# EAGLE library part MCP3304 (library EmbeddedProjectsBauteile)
Microchip 13-Bit Differential Input, Low Power A/D Converter with SPI Serial Interface
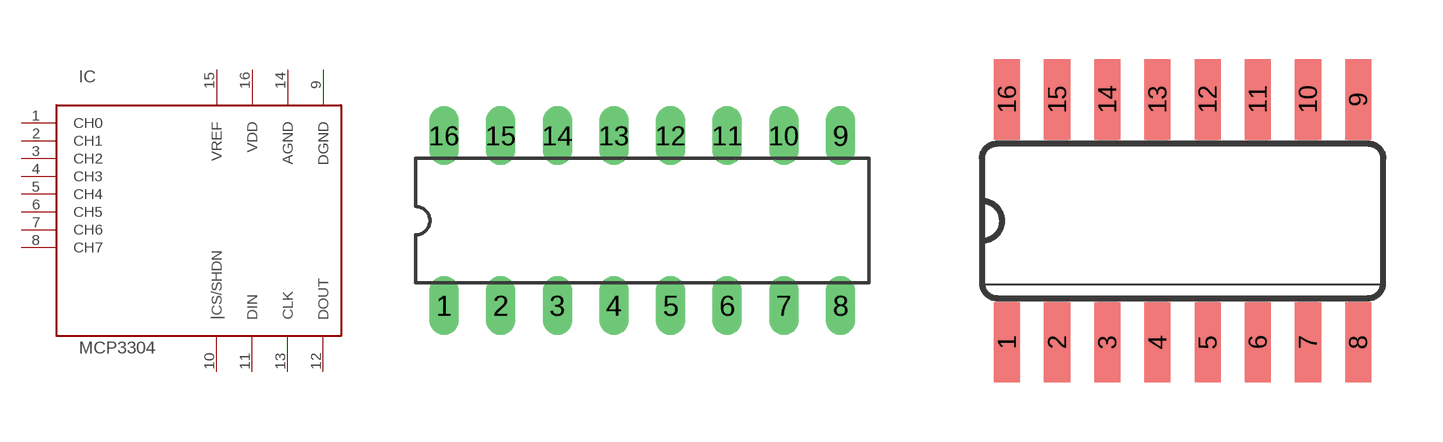
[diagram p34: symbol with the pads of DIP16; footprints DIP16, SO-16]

Designator prefix IC

## MCP3304BI/P (FARNELL: 1852025)  [DIP16]
1  CH0
2  CH1
3  CH2
4  CH3
5  CH4
6  CH5
7  CH6
8  CH7
9  DGND
10  |CS/SHDN
11  DIN
12  DOUT
13  CLK
14  AGND
15  VREF
16  VDD

## MCP3304BI/SL (EP: 401140; FARNELL: 1852026)  [SO-16]
Pads as for DIP16

## Footprint DIP16 (pad centres in mm)
drill 0.813 long: 1 -8.89,-3.81; 2 -6.35,-3.81; 3 -3.81,-3.81; 4 -1.27,-3.81; 5 1.27,-3.81; 6 3.81,-3.81; 7 6.35,-3.81; 8 8.89,-3.81; 9 8.89,3.81; 10 6.35,3.81; 11 3.81,3.81; 12 1.27,3.81; 13 -1.27,3.81; 14 -3.81,3.81; 15 -6.35,3.81; 16 -8.89,3.81

## Footprint SO-16 (pad centres in mm)
smd 0.66 x 2.032: 1 -4.445,-3.073; 2 -3.175,-3.073; 3 -1.905,-3.073; 4 -0.635,-3.073; 5 0.635,-3.073; 6 1.905,-3.073; 7 3.175,-3.073; 8 4.445,-3.073; 9 4.445,3.073; 10 3.175,3.073; 11 1.905,3.073; 12 0.635,3.073; 13 -0.635,3.073; 14 -1.905,3.073; 15 -3.175,3.073; 16 -4.445,3.073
